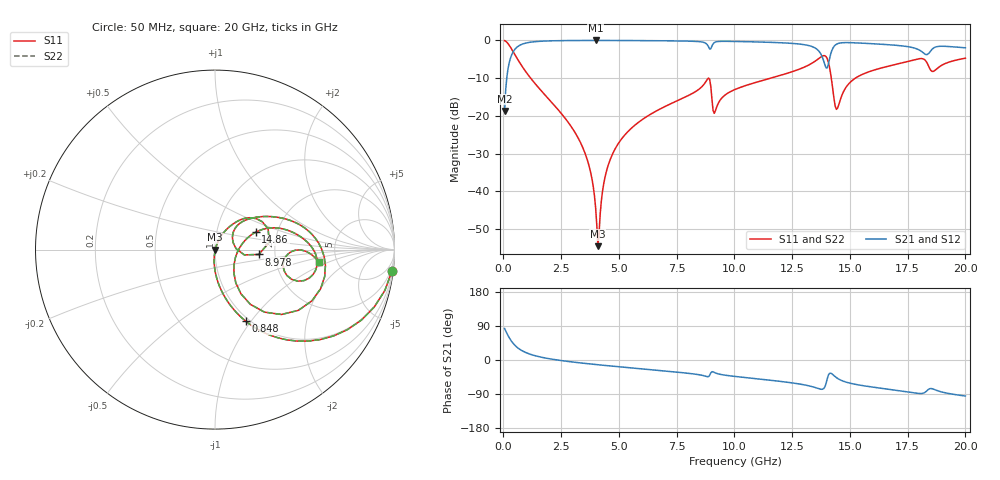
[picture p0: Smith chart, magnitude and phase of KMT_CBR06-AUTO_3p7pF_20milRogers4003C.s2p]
! Data measured by Modelithics Inc. support@modelithics.com 813-866-6335
! KEMET CBR06-AUTO 3.7pF, Pad Width= 0.851mm, Pad Length= 0.64mm, Pad Gap= 0.62mm, 20mil Rogers 4003C substrate Data, January 2022
# hz S ma R 50
! 2 Port Network Data from SP1.SP block
! freq  magS11  angS11  magS21  angS21  magS12  angS12  magS22  angS22
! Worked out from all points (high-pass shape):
!   401 points, 50 MHz to 20 GHz, reference 50 ohm
!   highest |S21| = -0.02 dB at 3.99 GHz (marker M1); lowest = -18.7 dB at 50 MHz (marker M2)
!   |S21| within 3 dB of the highest: 423.8 MHz to 13.68 GHz (13.25 GHz wide, 188 % of centre); 14.2 GHz to 18.12 GHz (3.921 GHz wide, 24.3 % of centre)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
!   lowest |S11| = -54.5 dB at 4.09 GHz (marker M3), VSWR 1.00, Z = 50.2 - j0.0886 ohm
!   |S11| at or under -10 dB: 1.177 GHz to 8.872 GHz (7.695 GHz wide, 153 % of centre); 8.883 GHz to 11.57 GHz (2.684 GHz wide, 26.2 % of centre); 14.19 GHz to 15.24 GHz (1.044 GHz wide, 7.09 % of centre)
!   |S22| runs from -54.5 to -0.1 dB; largest |S21 - S12| = 0
!   S11 on the Smith chart (normalised r, x): 50 MHz: 1, -17; 848 MHz: 0.96, -0.94; 8.978 GHz: 1.64, -0.10; 14.86 GHz: 1.55, +0.32; 20 GHz: 3.62, -0.73
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5e7  0.9932 -6.8  0.1164 83.1  0.1164 83.1  0.9932 -6.8
3.4925e8  0.7713 -40.5  0.6356 49.4  0.6356 49.4  0.7713 -40.5
8.48e8  0.4342 -66.7  0.8998 23.1  0.8998 23.1  0.4342 -66.7
3.391625e9  0.04079 -95.7  0.9974 -8.1  0.9974 -8.1  0.04079 -95.7
3.790625e9  0.01698 -94.7  0.998 -10.7  0.998 -10.7  0.01698 -94.7
3.990125e9  0.006113 -84.8  0.998 -11.9  0.998 -11.9  0.006113 -84.8
4.089875e9  0.001884 -28.0  0.998 -12.5  0.998 -12.5  0.001884 -28.0
4.439e9  0.01751 69.2  0.9978 -14.6  0.9978 -14.6  0.01751 69.2
4.838e9  0.03676 70.0  0.9972 -16.9  0.9972 -16.9  0.03676 70.0
6.73325e9  0.1214 61.3  0.9898 -27.5  0.9898 -27.5  0.1214 61.3
8.828e9  0.3057 30.5  0.8737 -44.0  0.8737 -44.0  0.3057 30.5
8.977625e9  0.2456 -6.4  0.7753 -33.8  0.7753 -33.8  0.2456 -6.4
9.177125e9  0.1172 34.0  0.9502 -34.2  0.9502 -34.2  0.1172 34.0
1.0025e10  0.2237 45.1  0.9684 -43.4  0.9684 -43.4  0.2237 45.1
1.336662e10  0.5006 15.3  0.8272 -70.3  0.8272 -70.3  0.5006 15.3
1.38155e10  0.6217 -8.3  0.5898 -77.1  0.5898 -77.1  0.6217 -8.3
1.406488e10  0.5177 -44.3  0.4824 -40.3  0.4824 -40.3  0.5177 -44.3
1.4414e10  0.122 -20.9  0.888 -46.4  0.888 -46.4  0.122 -20.9
1.486288e10  0.2471 23.2  0.9349 -58.9  0.9349 -58.9  0.2471 23.2
1.670825e10  0.4592 11.0  0.8751 -77.4  0.8751 -77.4  0.4592 11.0
1.830425e10  0.5253 -19.2  0.6481 -82.8  0.6481 -82.8  0.5253 -19.2
2e10  0.5812 -6.6  0.7979 -95.1  0.7979 -95.1  0.5812 -6.6
